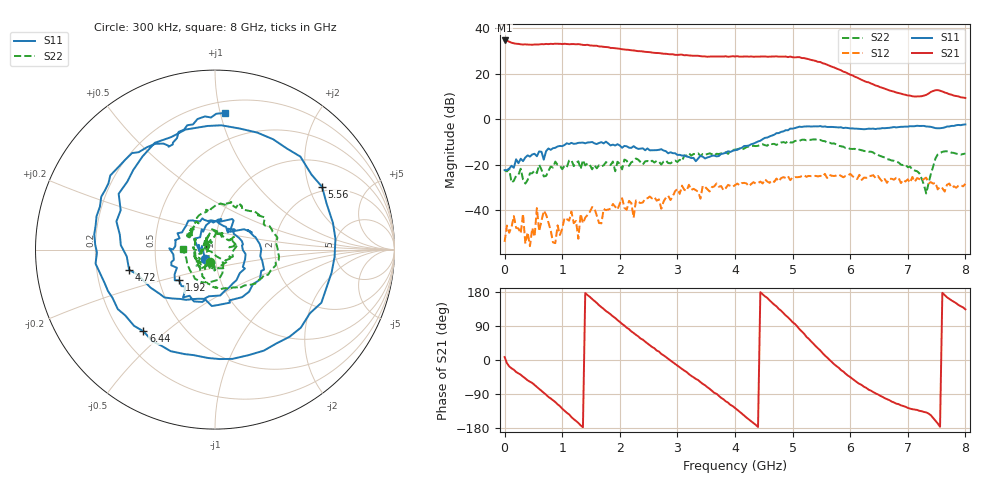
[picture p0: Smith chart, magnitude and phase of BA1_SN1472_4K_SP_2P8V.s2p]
! VC=2.8V IC=22.3mA
# HZ S DB R 50.00
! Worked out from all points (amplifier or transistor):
!   201 points, 300 kHz to 8 GHz, reference 50 ohm
!   highest |S21| = 34.5 dB at 300 kHz (marker M1)
!   |S21| within 3 dB of that: start of sweep to 1.803 GHz
!   unconditionally stable (mu >= 1): start of sweep to 2.996 GHz; 3.288 GHz to 3.433 GHz; 6.188 GHz to end of sweep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
!   at 1.32 GHz: K = 1.42, MAG = 33.3 dB, |S12| = -41.6 dB
!   at 4 GHz: K = 0.92, MSG = 28.2 dB, |S12| = -29.0 dB
!   at 8 GHz: K = 1.80, MAG = 13.6 dB, |S12| = -28.4 dB
!   S11 on the Smith chart (normalised r, x): 300 kHz: 0.89, -0.09; 1.92 GHz: 0.63, -0.23; 4.72 GHz: 0.35, -0.10; 5.56 GHz: 1.84, +2.46; 6.44 GHz: 0.29, -0.42; 8 GHz: 0.28, +1.03
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300000  -22.38 -136.8  34.51 7.9  -53.85 -143.4  -22.42 -112.7
8.0297e7  -21.72 -164.8  33.96 -17.0  -49.87 -151.6  -21.86 -173.2
2.002925e8  -17.62 152.8  33.07 -31.7  -47.72 -134.5  -24.84 154.3
7.20273e8  -14.08 35.0  32.99 -91.6  -41.86 122.9  -24.95 122.9
9.60264e8  -11.77 0.5  33.04 -121.7  -50.81 81.6  -20.34 69.5
1.200255e9  -10.86 -41.6  32.91 -156.2  -45.65 76.8  -20.62 31.9
1.360249e9  -10.31 -60.3  32.55 -177.6  -45.69 129.4  -17.98 10.9
1.640238e9  -10.45 -103.7  31.89 144.4  -45.59 48.8  -20.24 -43.5
1.920228e9  -11.59 -139.7  31.09 110.9  -38.46 -25.5  -22.88 -91.1
2.360212e9  -12.96 167.7  29.80 56.7  -36.82 -35.9  -18.85 -141.1
2.6802e9  -13.47 137.9  28.97 22.2  -35.23 -56.4  -18.64 -172.2
3.320176e9  -18.48 52.8  27.81 -49.9  -31.19 -100.6  -15.32 154.5
4.00015e9  -13.64 -54.8  27.48 -126.5  -28.96 -163.3  -13.39 110.4
4.400135e9  -9.82 -119.9  27.44 -176.8  -28.04 147.9  -11.72 79.0
4.720123e9  -6.17 -166.8  27.52 141.7  -26.09 120.4  -11.35 55.6
5.08011e9  -3.64 127.8  27.17 88.7  -25.50 82.2  -9.46 18.4
5.360099e9  -3.18 70.1  25.78 43.2  -25.03 54.0  -8.90 -6.0
5.560092e9  -3.20 30.3  24.28 12.1  -24.03 28.4  -9.70 -25.5
5.920078e9  -3.79 -42.3  20.53 -36.2  -24.96 -11.5  -12.67 -65.2
6.440058e9  -4.37 -131.2  14.76 -88.0  -25.82 -55.5  -15.38 -110.4
6.68005e9  -3.84 -163.4  12.60 -105.9  -26.17 -77.3  -17.76 -135.3
8e9  -2.35 85.9  9.24 133.7  -28.37 -174.5  -15.07 178.7
